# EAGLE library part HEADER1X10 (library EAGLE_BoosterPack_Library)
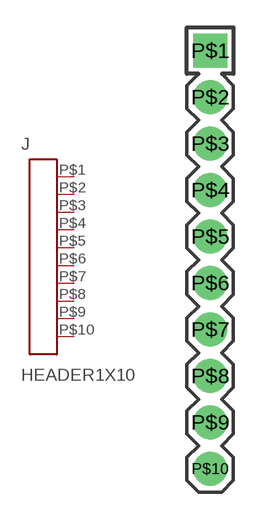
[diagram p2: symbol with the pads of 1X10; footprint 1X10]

Designator prefix J

## HEADER1X10  [1X10]
P$1  1
P$2  2
P$3  3
P$4  4
P$5  5
P$6  6
P$7  7
P$8  8
P$9  9
P$10  10

## Footprint 1X10 (pad centres in mm)
drill 1.016 pad 1.88 square: P$1 0,10.16
drill 1.016 pad 1.88: P$2 0,7.62; P$3 0,5.08; P$4 0,2.54; P$5 0,0; P$6 0,-2.54; P$7 0,-5.08; P$8 0,-7.62; P$9 0,-10.16; P$10 0,-12.7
